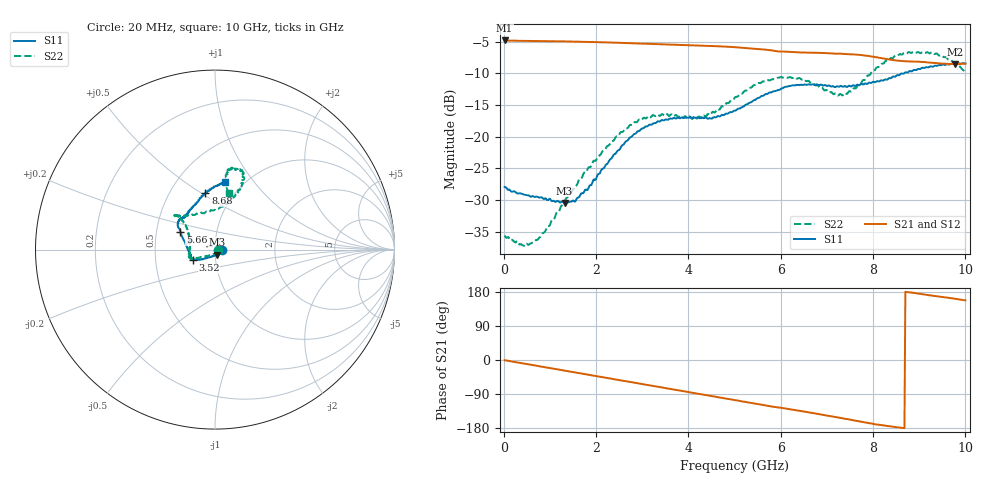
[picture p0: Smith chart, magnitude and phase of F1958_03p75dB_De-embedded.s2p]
! Integrated Device Technology
! Corporate Headquarters
! 6024 Silver Creek Valley Road
! San Jose, CA 95138  USA
! Phone:  1-408-284-8200
! Toll Free:  1-800-223-1366
! Webpage:  http://www.idt.com/
! Timing and RF Division
! 515 Groton Road, Suite 102
! Westford, MA 01886-6024
! Device:  F1958
! Description: 7-bit 0.25 dB Digital Step Attenuator
! Frequency:  0.001 -  6.000 GHz
! Package:  4x4 mm Thin QFN Plastic Package: 24 pin
! Ports:  2 RF, 12 DC
!  Pin  1  = D0
!  Pin  2  = VDD
!  Pin  3  = VMODE
!  Pin  4  = GND
!  Pin  5  = RF1  =  Port 1
!  Pin  6  = GND
!  Pin  7  = GND
!  Pin  8  = GND
!  Pin  9  = GND
!  Pin 10  = GND
!  Pin 11  = GND
!  Pin 12  = GND
!  Pin 13  = GND
!  Pin 14  = RF2  =  Port 2
!  Pin 15  = GND
!  Pin 16  = LE
!  Pin 17  = CLK
!  Pin 18  = DATA
!  Pin 19  = D6
!  Pin 20  = D5
!  Pin 21  = D4
!  Pin 22  = D3
!  Pin 23  = D2
!  Pin 24  = D1
! State:  15
! Atten State:  3.75 dB
! Voltage:  +3.30 Volts
! Current:  0.257 mA
! Data:  The device was measured on a F1958 evaluation board which has
!  individual transmission lines to the RF pins.  Data was collected
!  using a calibrated network analyzer.  The evaluation board was
!  de-embedded using Automatic Fixture Removal (AFR).
!  The reference plane is the edge of the package pin.
! Misc:
!  Action Tracker AT0419
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# GHz S dB R 50
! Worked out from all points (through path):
!   500 points, 20 MHz to 10 GHz, reference 50 ohm
!   highest |S21| = -4.78 dB at 20 MHz (marker M1); lowest = -8.5 dB at 9.78 GHz (marker M2)
!   group delay of S21, straight-line fit = 57.1 ps
!   lowest |S11| = -30.5 dB at 1.32 GHz (marker M3), VSWR 1.06, Z = 51.2 - j2.8 ohm
!   |S11| at or under -10 dB: start of sweep to 8.618 GHz; 8.622 GHz to 8.668 GHz (45.88 MHz wide, 0.531 % of centre)
!   |S22| runs from -37.3 to -6.6 dB; largest |S21 - S12| = 0.0016
!   S11 on the Smith chart (normalised r, x): 20 MHz: 1.08, -0.00; 3.52 GHz: 0.77, -0.09; 5.66 GHz: 0.67, +0.14; 8.68 GHz: 0.74, +0.52; 10 GHz: 0.83, +0.72
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0.02  -27.93 -3.0  -4.78 -0.6  -4.79 -0.5  -35.61 -7.4
0.42  -29.09 -11.9  -4.85 -9.0  -4.85 -9.0  -37.17 -34.9
0.64  -29.40 -19.0  -4.87 -13.6  -4.86 -13.6  -36.67 -55.4
0.9  -29.71 -32.0  -4.89 -19.1  -4.88 -19.1  -34.92 -82.5
1.32  -30.47 -65.7  -4.93 -28.1  -4.93 -28.1  -30.25 -118.0
1.52  -30.14 -82.6  -4.97 -32.3  -4.96 -32.3  -28.08 -128.6
1.7  -28.91 -97.1  -4.99 -36.0  -4.99 -36.0  -26.37 -136.3
2.58  -21.30 -141.2  -5.18 -54.6  -5.16 -54.6  -19.22 -154.4
2.94  -19.06 -149.0  -5.27 -62.2  -5.26 -62.3  -17.28 -157.8
3.36  -17.58 -153.6  -5.38 -71.0  -5.38 -71.1  -16.61 -161.8
3.52  -17.25 -154.8  -5.41 -74.3  -5.42 -74.4  -16.44 -166.0
4.32  -17.04 -165.5  -5.59 -91.1  -5.61 -91.2  -16.65 166.2
5.02  -15.87 172.1  -5.85 -106.0  -5.86 -106.0  -13.72 141.8
5.66  -13.32 153.1  -6.23 -119.5  -6.24 -119.5  -11.30 137.7
6.18  -11.98 145.7  -6.58 -129.5  -6.59 -129.5  -10.61 139.1
6.68  -11.72 139.5  -6.72 -139.5  -6.74 -139.4  -11.50 134.3
7.38  -12.01 130.5  -6.91 -154.7  -6.92 -154.6  -13.10 95.9
8.34  -10.76 108.5  -7.78 -174.8  -7.78 -174.9  -7.89 67.2
8.68  -9.93 99.6  -8.07 -179.8  -8.07 -179.7  -6.73 70.6
9.3  -8.91 86.9  -8.31 169.4  -8.31 169.4  -6.79 80.3
9.78  -8.43 82.5  -8.52 161.6  -8.54 161.6  -8.31 80.4
10  -8.44 81.8  -8.46 157.3  -8.49 157.4  -9.79 76.4
